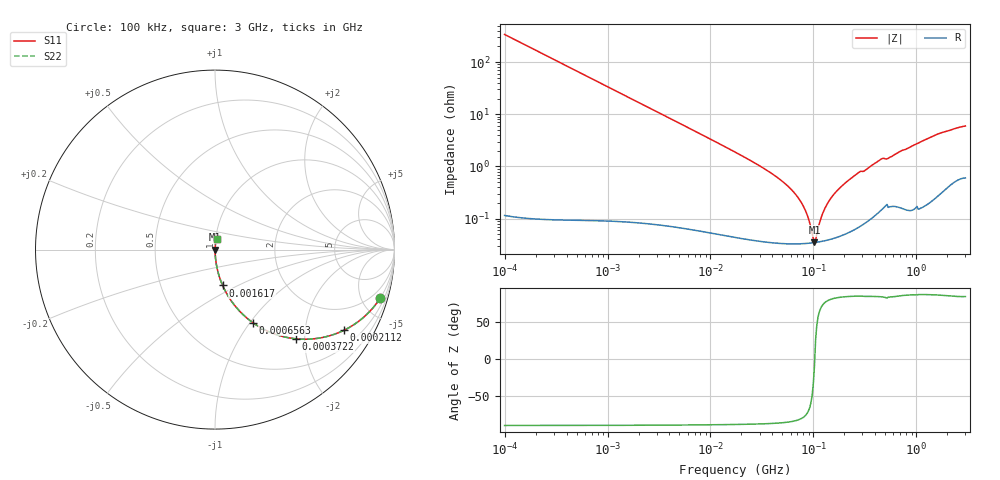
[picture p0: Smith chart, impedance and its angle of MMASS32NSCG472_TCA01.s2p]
! MMASS32NSCG472_TCA01  S-PARAMETER MODEL  ( Standard Model )
! Model Generated by TAIYO YUDEN Corporation (https://www.yuden.co.jp/en/)
! Version 1.0
! TAIYO YUDEN Control No. 250312
! Copyright(c) 2025 TAIYO YUDEN CO.,LTD. All Rights Reserved.
! Product Description (link to TY-COMPAS)
! https://ds.yuden.co.jp/TYCOMPAS/or/detail?pn=MMASS32NSCG472JTCA01&u=M
! Products Name : Multilayer Ceramic Capacitors
! Characteristics :
!  Capacitance : 4700 [pF] , Rated Voltage : 630 [V] , TCC : CG / C0G
!  Case Size : 3.2 x 2.5 / 0.126 x 0.098 [mm/inch] , Thickness : 1.9 / 0.075 [mm/inch]
!  (Conditions: Temperature = 25 [degC] , DC Bias Voltage = 0 [V])
! External Node Assignments :
!  1  o---| |---o  2
! GND o---------o GND
! Frequency Range : 0.1MHz  -  3000MHz  [ 401 STEP ]
# MHZ S RI R 50
! Freq[MHz].  S11 Real  S11 Imag  S21 Real  S21 Imag  S12 Real  S12 Imag  S22 Real  S22 Imag
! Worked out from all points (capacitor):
!   401 points, 100 kHz to 3 GHz, reference 50 ohm
!   read as one part in series: C = 4.72 nF near 105.3 kHz
!   lowest |Z| = 35.3 mohm at 102.5 MHz (marker M1)
!   series resonance near 103.2 MHz, so ESL is about 500 pH
!   S11 on the Smith chart (normalised r, x): 100 kHz: 1.00, -6.75; 211.2 kHz: 1.00, -3.20; 372.2 kHz: 1.00, -1.81; 656.3 kHz: 1.00, -1.03; 1.617 MHz: 1.00, -0.42; 3 GHz: 1.01, +0.12
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0.1  0.9192 -0.2724  0.0808 0.2724  0.0808 0.2724  0.9192 -0.2724
0.21115  0.7185 -0.4494  0.2815 0.4494  0.2815 0.4494  0.7185 -0.4494
0.372249  0.4513 -0.4971  0.5487 0.4971  0.5487 0.4971  0.4513 -0.4971
0.562235  0.2654 -0.4408  0.7346 0.4408  0.7346 0.4408  0.2654 -0.4408
0.656258  0.2098 -0.4062  0.7902 0.4062  0.7902 0.4062  0.2098 -0.4062
1.61742  0.0425 -0.1997  0.9575 0.1997  0.9575 0.1997  0.0425 -0.1997
3.161081  0.012 -0.1053  0.988 0.1053  0.988 0.1053  0.012 -0.1053
17.7727  0.000771 -0.0184  0.9992 0.0184  0.9992 0.0184  0.000771 -0.0184
38.50681  0.000404 -0.00754  0.9996 0.00754  0.9996 0.00754  0.000404 -0.00754
61.23616  0.000341 -0.00358  0.9997 0.00358  0.9997 0.00358  0.000341 -0.00358
81.30716  0.000335 -0.00159  0.9997 0.00159  0.9997 0.00159  0.000335 -0.00159
90.13636  0.000339 -0.000902  0.9997 0.000902  0.9997 0.000902  0.000339 -0.000902
97.38194  0.000344 -0.000394  0.9997 0.000394  0.9997 0.000394  0.000344 -0.000394
102.5331  0.000348 -5.66e-05  0.9997 5.66e-05  0.9997 5.66e-05  0.000348 -5.66e-05
107.9567  0.000354 0.000354  0.9996 -0.000354  0.9996 -0.000354  0.000354 0.000354
129.3002  0.00038 0.00152  0.9996 -0.00152  0.9996 -0.00152  0.00038 0.00152
167.3121  0.000446 0.00329  0.9996 -0.00329  0.9996 -0.00329  0.000446 0.00329
273.0175  0.000732 0.00752  0.9993 -0.00752  0.9993 -0.00752  0.000732 0.00752
457.1373  0.00165 0.0138  0.9984 -0.0138  0.9984 -0.0138  0.00165 0.0138
547.5153  0.00189 0.0147  0.9981 -0.0147  0.9981 -0.0147  0.00189 0.0147
1575.075  0.00422 0.0406  0.9958 -0.0406  0.9958 -0.0406  0.00422 0.0406
3000  0.00944 0.0585  0.9906 -0.0585  0.9906 -0.0585  0.00944 0.0585
